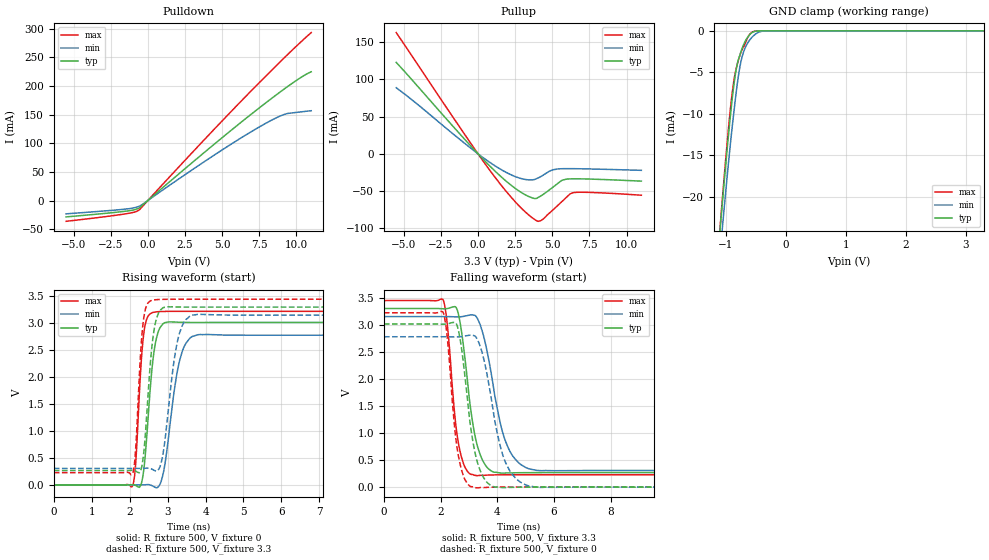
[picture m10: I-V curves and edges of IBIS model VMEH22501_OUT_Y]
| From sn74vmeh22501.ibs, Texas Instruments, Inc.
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[Model]   VMEH22501_OUT_Y
Model_type  3-state
Enable   Active-Low
Vref =   0
Rref =   500
Cref =   50p
Vmeas =   1.5
| variable   typ   min   max
C_comp   3.15pF   2.68pF   3.83pF
| C_pullup   2.44pF   1.68pF   3.86pF
| C_pulldown   1.87pF   1.55pF   2.43pF
| C_tri-state   3.15pF   2.68pF   3.83pF
[Temperature Range]   40   100   0
| Ambient temperature   25   85   0
[Voltage range]   3.3   3.15   3.45
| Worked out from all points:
|   slope of the pulldown table from 0 to 0.495 V, typ, clamps not added: 44.2 ohm
|   slope of the pullup table from 0 to 0.495 V, typ, clamps not added: 47.8 ohm
|   GND clamp passes 1 mA (typ) near -0.66 V on its own axis
|   rising waveform, R_fixture 500, V_fixture 0: 20-80 % time 213ps typ, 325ps min, 157ps max; typ from 0.001 V to 3.01 V
|   falling waveform, R_fixture 500, V_fixture 3.3: 20-80 % time 459ps typ, 661ps min, 336ps max; typ from 3.3 V to 0.268 V
|   rising waveform, R_fixture 500, V_fixture 3.3: 20-80 % time 201ps typ, 298ps min, 151ps max; typ from 0.268 V to 3.3 V
|   falling waveform, R_fixture 500, V_fixture 0: 20-80 % time 451ps typ, 634ps min, 337ps max; typ from 3.01 V to 0.001 V
[GND Clamp]
| VMEH22501_OUT_Y
|   Voltage   I(typ)   I(min)   I(max)
-5.5V     -441.1mA   -423.7mA   -468.4mA
-1.095V   -23.52mA   -26.45mA   -23.26mA
-1.07V    -21.42mA   -24.45mA   -21.02mA
-1.045V   -19.35mA   -22.46mA   -18.82mA
-925mV    -10.06mA   -13.45mA   -9.23mA
-875mV    -6.844mA   -10.15mA   -6.276mA
-825mV    -4.437mA   -7.076mA   -4.367mA
-770mV    -2.956mA   -4.392mA   -2.974mA
-710mV    -1.72mA    -2.599mA   -1.943mA
-610mV    -495.1uA   -1.154mA   -475.8uA
-510mV    -53.25uA   -403.4uA   -34.88uA
3.3V      93.06pA    4.492nA    -730.5pA
[Pulldown]
| VMEH22501_OUT_Y
|   Voltage   I(typ)   I(min)   I(max)
-5.5V     -28.59mA   -23.27mA   -36.27mA
-1.64V    -19.09mA   -15.32mA   -23.8mA
-905mV    -16.16mA   -12.58mA   -20.27mA
-600mV    -13.19mA   -10.16mA   -16.81mA
4.645V    102.1mA    82.34mA    129.3mA
6.435V    139.9mA    111.9mA    177.7mA
7.895V    169.7mA    134.3mA    216.1mA
8.73V     186.2mA    145.5mA    237.7mA
9.305V    197.2mA    151.4mA    252.4mA
10.34V    215.5mA    155mA      277.8mA
11V       224.9mA    156.9mA    293.4mA
[Pullup]
| VMEH22501_OUT_Y
|   Voltage   I(typ)   I(min)   I(max)
-5.5V     122.7mA    88.67mA    162.8mA
-960mV    20.9mA     15.05mA    27.94mA
1.005V    -20.53mA   -14.36mA   -27.75mA
2.64V     -48.35mA   -31.65mA   -67.32mA
3.285V    -56.16mA   -34.82mA   -79.95mA
3.83V     -60.17mA   -34.4mA    -88.47mA
4.06V     -58.62mA   -32.42mA   -90.76mA
4.315V    -55.68mA   -29.67mA   -88.82mA
4.965V    -46.2mA    -22.17mA   -77mA
5.645V    -35.95mA   -20.12mA   -64.41mA
6.415V    -33.68mA   -20.06mA   -52.34mA
11V       -36.8mA    -22.29mA   -55.73mA
[Ramp]
| VMEH22501_OUT_Y
| variable   typ   min   max
dV/dt_r   1.84/2.21E-10   1.71/3.43E-10   1.95/1.61E-10
dV/dt_f   1.84/4.80E-10   1.72/6.93E-10   1.95/3.48E-10
R_load = 500
[Rising Waveform]
| VMEH22501_OUT_Y
R_fixture =   500
C_fixture =   0
L_fixture =   0
V_fixture =   0
V_fixture_min = 0
V_fixture_max = 0
|   Time   V(typ)   V(min)   V(max)
0s        762.1uV    2.362uV    2.723mV
2.08ns    5.113mV    -55.12uV   -14.85mV
2.155ns   -7.895mV   -194.1uV   375mV
2.29ns    -6.424mV   -23.52uV   2.127V
2.37ns    272.2mV    1.368mV    2.798V
2.665ns   2.579V     -41.35mV   3.207V
2.895ns   2.998V     249.1mV    3.217V
3.34ns    3.017V     2.367V     3.22V
3.81ns    3.014V     2.787V     3.22V
24.99ns   3.014V     2.777V     3.22V
[Falling Waveform]
| VMEH22501_OUT_Y
R_fixture =   500
C_fixture =   0
L_fixture =   0
V_fixture =   3.3
V_fixture_min = 3.15
V_fixture_max = 3.45
|   Time   V(typ)   V(min)   V(max)
0s        3.299V     3.15V      3.447V
2.085ns   3.294V     3.15V      3.466V
2.235ns   3.299V     3.15V      3.012V
2.63ns    3.192V     3.144V     811.3mV
2.87ns    2.332V     3.16V      357.3mV
3.21ns    958.3mV    3.173V     217.6mV
3.625ns   373.7mV    2.55V      220.7mV
4.275ns   259.6mV    871.1mV    227.6mV
5.15ns    267mV      333.7mV    228.1mV
24.99ns   267.7mV    306.2mV    227.9mV
[Rising Waveform]
| VMEH22501_OUT_Y
R_fixture =   500
C_fixture =   0
L_fixture =   0
V_fixture =   3.3
V_fixture_min = 3.15
V_fixture_max = 3.45
|   Time   V(typ)   V(min)   V(max)
0s        267.8mV    306.2mV    228.1mV
2.08ns    272.2mV    306.2mV    214.1mV
2.155ns   259.4mV    306.1mV    640.8mV
2.275ns   246mV      306.1mV    2.287V
2.355ns   503.9mV    307.4mV    3.008V
2.62ns    2.765V     280.2mV    3.429V
2.865ns   3.279V     524.8mV    3.441V
3.29ns    3.3V       2.754V     3.444V
3.66ns    3.298V     3.151V     3.444V
24.99ns   3.299V     3.15V      3.446V
[Falling Waveform]
| VMEH22501_OUT_Y
R_fixture =   500
C_fixture =   0
L_fixture =   0
V_fixture =   0
V_fixture_min = 0
V_fixture_max = 0
|   Time   V(typ)   V(min)   V(max)
0s        3.014V     2.778V     3.22V
2.085ns   3.01V      2.778V     3.235V
2.23ns    3.015V     2.778V     2.79V
2.475ns   3.043V     2.775V     1.215V
2.61ns    2.937V     2.775V     632.5mV
3.08ns    1.04V      2.807V     8.147mV
3.495ns   195.3mV    2.428V     -8.422mV
4.25ns    -9.081mV   510.9mV    2.099mV
5.105ns   -119.6uV   23.12mV    2.659mV
24.99ns   725.6uV    2.413uV    2.548mV
